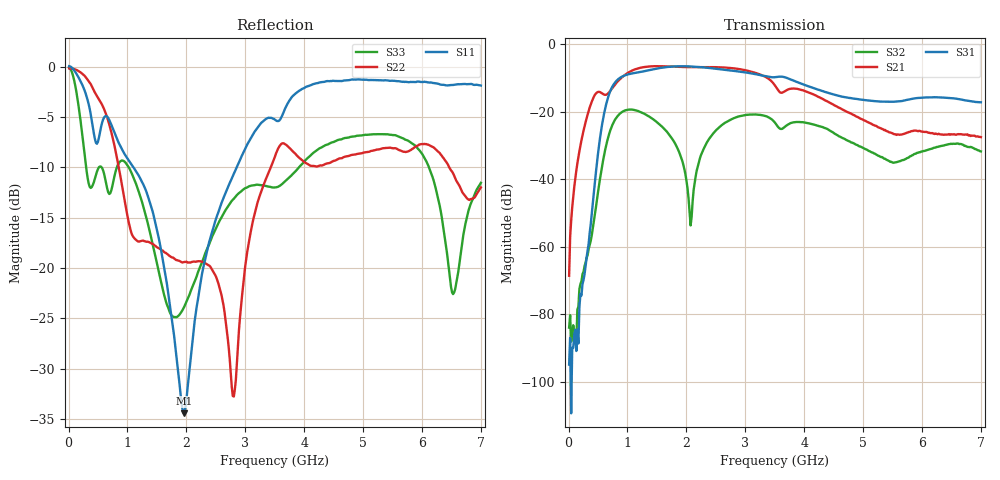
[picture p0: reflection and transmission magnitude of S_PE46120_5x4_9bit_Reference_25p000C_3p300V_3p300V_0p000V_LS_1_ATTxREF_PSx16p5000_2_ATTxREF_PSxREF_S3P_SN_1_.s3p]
! Device ID: PE46120_5x4_9bit_Reference
! Device ID: PE46120_5x4_9bit_Reference
! File Path: z:\PE46120_5x4_9bit_Reference\MPAC_Yi\new_12port\25p000C\3p300\LS_1_ATTxREF_PSx16p5000_2_ATTxREF_PSxREF\PE46120_5x4_9bit_Reference_25p000C_3p300V_3p300V_0p000V_LS_1_ATTxREF_PSx16p5000_2_ATTxREF_PSxREF_S3P_SN_1_.s3p
! Serial: 1
! Lot:
! Temp: 25.000C
! VDD: 3.300
! VSS: 0.000
! Control_Hi: 3.300
! Control_Lo: 0.000
! Logic State: LS_1_ATTxREF_PSx16p5000_2_ATTxREF_PSxREF
! Port 1: RFin
! Port 2: RFout1
! Port 3: RFout2
! ThroughPath:1-2
! IDD: -0.0005485403
! ISS: 0
! Comment:
#  Hz  S  RI  R  50
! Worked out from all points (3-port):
!   401 points, 10 MHz to 7 GHz, reference 50 ohm
!   strongest paths, dB at 10 MHz, 1.758 GHz, 3.505 GHz, 5.253 GHz, 7 GHz:
!     S31: -94.8, -6.7, -9.8, -17.0, -17.2
!     S21: -68.5, -6.7, -12.3, -24.6, -27.6
!     S32: -83.9, -28.0, -23.3, -33.0, -31.8
!   lowest |S11| = -34.4 dB at 1.967 GHz (marker M1), VSWR 1.04, Z = 51.9 + j0.418 ohm
!   |S11| at or under -10 dB: 1.104 GHz to 2.851 GHz (1.747 GHz wide, 88.4 % of centre)
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1e7  1.002 -0.1146  4.83e-05 0.000337  -7.23e-05 -3.89e-05
     7.42e-05 0.000367  0.9838 -0.0309  -3.7e-05 2.39e-05
     -1.81e-05 1.12e-06  4.96e-05 4.05e-05  0.9882 -0.0962
3.07075e8  -0.6131 -0.3625  -0.0122 0.0781  0.000452 0.000397
           -0.0123 0.0789  0.5121 -0.7114  -0.000523 0.000487
           0.000571 0.000404  -0.000532 0.000432  -0.303 -0.0154
5.692e8  -0.5185 -0.0955  0.1813 0.0337  0.0449 -0.045
         0.1833 0.034  -0.1057 -0.6398  0.0154 -0.000278
         0.0452 -0.0454  0.0155 -0.000141  0.3141 0.0161
8.31325e8  -0.3647 0.232  0.2568 -0.0952  -0.2648 0.1231
           0.26 -0.0969  -0.2871 -0.1852  -0.0759 0.0371
           -0.2678 0.1251  -0.0767 0.0378  0.2513 -0.2028
1.37305e9  -0.0702 0.2038  -0.3117 -0.3369  0.4015 -0.0595
           -0.3162 -0.3408  -0.1287 -0.0382  -0.00604 -0.083
           0.4058 -0.0609  -0.00628 -0.0838  -0.1456 -0.0516
1.9672e9  0.0185 0.00403  -0.2569 0.3691  -0.2649 -0.3796
          -0.2598 0.3742  -0.0329 0.1021  0.00466 0.013
          -0.2687 -0.3833  0.0049 0.0131  -0.0644 -0.000582
2.07205e9  0.028 -0.0211  -0.1408 0.4262  -0.3684 -0.2754
           -0.1419 0.4318  0.00444 0.1064  0.0018 -0.00102
           -0.3735 -0.2776  0.00187 -0.000894  -0.0759 0.00956
2.806e9  -0.0476 -0.2909  0.4206 -0.0942  -0.0935 0.3843
         0.426 -0.0965  -0.0111 -0.0201  0.043 0.0663
         -0.0936 0.3892  0.0435 0.067  0.0657 0.211
3.505e9  -0.4458 -0.3153  -0.1785 -0.1598  0.311 0.0676
         -0.1812 -0.1619  0.2245 0.2795  -0.0324 -0.0597
         0.3154 0.0681  -0.0329 -0.0602  0.1783 -0.1774
7e9  -0.1104 0.8004  -0.0369 -0.018  0.1234 0.055
     -0.0378 -0.0182  -0.1683 0.1872  0.025 -0.00365
     0.1257 0.0552  0.0256 -0.00329  0.1483 0.2199
